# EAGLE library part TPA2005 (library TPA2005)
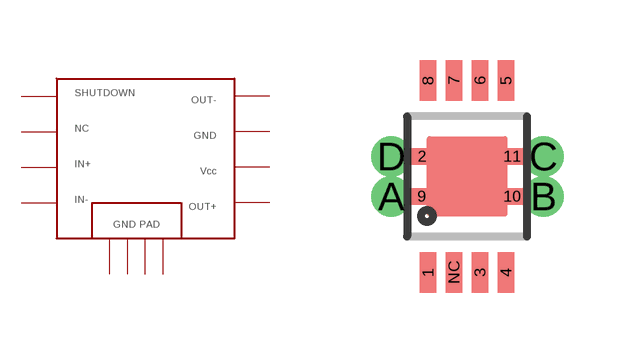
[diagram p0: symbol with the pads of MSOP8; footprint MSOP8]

Designator prefix -

## TPA2005  [MSOP8]
1  P$1
3  P$3
4  P$4
5  P$5
6  P$6
7  P$7
8  P$8
A  P$9
B  P$10
C  P$11
D  P$12
NC  P$2

## Footprint MSOP8 (pad centres in mm)
smd 0.41 x 1.02: 1 -0.975,-2.4; 3 0.325,-2.4; 4 0.975,-2.4; 5 0.975,2.4; 6 0.325,2.4; 7 -0.325,2.4; 8 -0.975,2.4; NC -0.325,-2.4
smd 1.02 x 0.41: 2 -1.13,0.5; 9 -1.13,-0.5; 10 1.13,-0.5; 11 1.13,0.5
drill 0.5 pad 0.813: A -1.9,-0.5; B 1.91,-0.5; C 1.91,0.5; D -1.9,0.5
